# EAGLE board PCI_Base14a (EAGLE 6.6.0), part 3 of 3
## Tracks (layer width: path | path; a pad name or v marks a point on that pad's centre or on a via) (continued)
V33  (via drill 0.3) (continued)
  Top 0.152: C14.1 76.99,5.54 83.34,11.89 83.66,11.89 | R4.2 59.21,24.59 65.72,31.1 74.77,31.1 X5.5
  Top 0.254: v47.94,82.06 47.62,82.38 v47.62,88.25 47.62,90.48 47.15,90.95 47.15,92.06 46.67,92.54 46.67,94.29 46.59,94.36 | v45.08,82.06 45.08,79.05 X2.A53 | 46.59,94.36 45.08,95.87 45.08,96.67 X2.A39 | v46.67,103.49 v46.67,101.11 46.67,94.44 46.59,94.36 | v55.72,100.95 55.72,104.92 57.63,106.83 58.42,106.83 58.74,107.14 59.21,107.14 59.37,106.99 60.48,106.99 X1.B31 | v49.69,111.11 50.01,110.8 v50.01,100.95 | v50.96,118.73 50.96,111.43 v51.28,111.11 | v14.45,77.62 v14.45,91.59 v14.45,100.48 14.45,103.33 14.76,103.65 14.76,110 14.45,110.32 v14.45,114.45 | X3.B41 19.37,94.13 19.37,91.75 X3.B43 | X3.A53 24.45,79.05 24.45,80.79 26.03,82.38 v26.03,88.25 26.51,88.73 26.51,93.33 26.03,93.81 26.03,97.62 | 20.64,111.59 20.64,112.38 19.37,113.65 19.37,114.45 X3.B25 | 20.64,111.59 20.64,108.89 19.37,107.62 19.37,106.99 X3.B31 | 26.03,97.62 24.76,97.62 24.45,97.3 24.45,96.83 X3.A39 | 26.03,103.49 26.03,97.62 | v33.5,103.49 v33.5,100.48 | 26.03,103.49 26.19,103.65 26.19,110.95 v25.88,111.27 26.19,111.11 26.19,115.4 26.03,115.56 v26.03,118.73 | 26.03,103.49 v25.88,103.65 | X2.B25 40,114.45 40,113.65 38.73,112.38 38.73,108.89 40,107.62 40,106.99 X2.B31 40,106.83 40,106.03 38.73,104.76 38.73,102.54 37.46,101.27 37.46,100.64 X2.B36 37.46,100.48 37.46,99.68 38.73,98.41 38.73,96.19 40,94.92 40,94.29 X2.B41 40,94.13 40,91.75 X2.B43 40,91.59 40,91.27 41.75,91.27 42.07,91.59 43.02,91.59 43.34,91.27 43.5,91.27 45.08,89.68 45.08,89.21 X2.A45 | 20.64,111.59 21.11,111.59 21.43,111.91 22.38,111.91 22.7,112.22 24.45,112.22 24.45,112.07 X3.A27 | 83.66,9.83 X7.1 | 83.66,13.96 X7.2
  Top 0.254: v80.96,13.96 v80.96,31.26 80.96,52.38 v81.28,52.69 | v96.84,119.21 v96.84,116.19 96.52,115.88 v96.52,109.21 v96.52,108.26 96.52,101.43 v96.88,101.15 | v80.8,101.11 80.8,105.91 v81.12,106.23 | v85.09,119.21 85.09,118.57 84.93,118.42 84.93,114.61 v85.25,114.21 84.93,114.45 84.93,111.59 v85.25,111.27 | 67.87,103.73 67.63,103.97 v67.63,104.29 | 67.87,103.73 68.1,103.49 v68.1,96.67 68.42,96.67 68.42,89.36 v68.26,89.05 | v67.31,119.53 v67.31,111.91 67.31,109.84 67.94,109.21 67.94,103.81 67.87,103.73 | X1.B41 60.64,94.13 60.64,91.75 X1.B43 60.64,91.59 60.64,90.79 62.07,89.36 v62.07,89.21 | v74.77,89.05 74.77,84.28 JP1.1 | v73.34,84.13 v73.34,78.89 v73.34,75.08 v73.34,62.85 | v83.03,62.54 83.34,62.22 83.34,59.36 83.82,58.88 C10.+ 83.82,57.77 v83.82,52.69 | X1.B54 58.1,77.62 58.1,77.14 60.17,75.08 60.96,75.08 61.91,76.03 62.39,76.03 62.71,76.35 63.5,76.35 65.72,78.57 65.72,78.89 X1.A53
  Top 0.813: 83.66,13.96 83.66,11.89 83.66,9.83
  Bottom 0.152: X6.J3-D8 87.36,101.11 v80.8,101.11 | X6.J3-A17 arc90 X6.J3-A17 v96.84,119.21 | X6.J3-A12 arc90 X6.J3-A12 v96.52,109.21 | X6.J3-B11 91.99,108.02 arc-90 92.55,108.26 v96.52,108.26 | X6.J3-A8 arc90 93.46,101.11 v96.88,101.15 | X6.J3-C14 89.36,114.03 arc19 88.87,114.12 arc71 88.63,114.21 v85.25,114.21 | X6.J3-C10 89.36,105.94 arc19 89.35,106.02 arc71 89.11,106.19 81.28,106.23 | X6.J3-D17 arc-90 X6.J3-D17 v85.09,119.21 | X6.J3-B15 91.36,115.94 arc-90 91.61,116.19 v96.84,116.19
  Bottom 0.203: X6.J3-D13 85.25,111.21 80.01,111.21 80.01,111.27
  Bottom 0.254: X2.A53 45.08,78.89 46.04,78.89 47.78,77.14 56.67,77.14 57.15,77.62 57.94,77.62 X1.B54 | v47.62,88.25 47.31,88.57 46.51,88.57 46.04,89.05 45.08,89.05 X2.A45 | v45.08,82.06 v47.94,82.06 | v46.67,103.49 46.67,103.65 46.04,104.29 45.08,104.29 X2.A33 | 55.8,101.03 55.56,101.27 51.59,101.27 51.43,101.11 51.28,101.11 51.12,101.27 50.01,101.27 | 55.8,101.03 56.36,100.48 57.94,100.48 X1.B36 | 50.01,101.27 46.83,101.27 v46.67,101.11 | v55.72,100.95 55.8,101.03 | 50.01,101.27 v50.01,100.95 | X2.A27 45.08,111.91 46.04,111.91 46.51,111.43 49.37,111.43 v49.69,111.11 v51.28,111.11 | v50.96,118.73 50.64,119.05 46.51,119.05 46.04,119.53 45.08,119.53 X2.A21 | v14.45,77.62 16.67,77.62 X3.B54 | v14.45,91.59 19.21,91.59 X3.B43 | v14.45,100.48 16.67,100.48 X3.B36 | X3.A53 24.45,78.89 25.4,78.89 25.88,78.41 35.4,78.41 36.19,77.62 37.31,77.62 X2.B54 | v26.03,88.25 26.03,88.41 25.4,89.05 24.45,89.05 X3.A45 | 25.88,103.81 25.4,104.29 24.45,104.29 X3.A33 | v33.5,100.48 37.31,100.48 X2.B36 | v33.5,103.49 33.18,103.81 25.88,103.81 | 25.88,103.81 v25.88,103.65 | v25.88,111.27 25.88,111.43 25.4,111.91 24.45,111.91 X3.A27 | v26.03,118.73 26.03,118.89 25.4,119.53 24.45,119.53 X3.A21 | v14.45,114.45 19.21,114.45 X3.B25 | 74.93,31.26 X5.5 | 83.5,13.96 X7.2 | 89.06,9.83 X7.11 | 83.66,9.83 X7.1 | X6.J3-B15 91.28,115.08 90.96,114.76 90.49,114.76 89.85,114.13 89.38,114.13 88.87,114.12 | X6.J3-B11 91.28,107.14 90.8,107.14 89.69,106.03 89.38,106.03 89.35,106.02 | 81.28,106.23 v81.12,106.23 | v85.25,111.27 85.25,111.21 | v68.1,96.67 65.72,96.67 X1.A39 | v67.63,104.29 65.72,104.29 X1.A33 | v67.31,119.53 65.72,119.53 X1.A21
  Bottom 0.254: X1.B25 60.64,114.45 61.12,114.45 61.59,113.97 61.59,112.7 61.91,112.7 62.71,111.91 65.56,111.91 X1.A27 65.72,111.91 v67.31,111.91 67.79,111.43 73.5,111.43 73.82,111.75 79.53,111.75 80.01,111.27 | v74.77,89.05 v68.26,89.05 65.72,89.05 X1.A45 65.56,89.05 62.71,89.05 62.55,89.21 v62.07,89.21 | v73.34,75.08 74.93,75.08 JP3.1 | v73.34,84.13 74.77,84.13 JP1.1 | v83.03,62.54 73.66,62.54 v73.34,62.85 | v73.34,78.89 65.72,78.89 X1.A53 | v83.82,52.69 v81.28,52.69
  Bottom 0.813: v80.96,31.26 74.93,31.26 | 83.5,13.96 v80.96,13.96 | 83.66,9.83 89.06,9.83
V33IO  (via drill 0.3)
  Top 0.254: v73.02,113.97 73.02,115.56 C16.1 | v77.31,113.97 77.31,84.28 JP1.2
  Bottom 0.254: v77.31,113.97 v73.02,113.97
VIO  (via drill 0.3)
  Top 0.254: v83.03,124.25 v83.03,131.12 83.03,138.58 83.34,138.89 83.34,144.61 83.03,144.93 v83.03,147.47 | v95.57,136.2 v95.57,147.31 | v29.05,65.08 29.05,63.65 R6.2 | v49.37,65.08 49.37,63.65 R5.2 | JP3.2 77.63,74.92 77.63,72.54 JP3.4 77.63,72.38 v77.63,65.87 | v98.42,75.08 98.42,79.36 C17.1 98.42,79.52 v98.42,89.05 v98.42,98.25 | v97.63,136.2 97.31,135.88 97.31,129.69 97.63,129.37 97.63,127.78 96.04,126.19 96.04,111.43 95.73,111.11 95.73,106.19 96.04,105.87 96.04,98.57 v96.36,98.17
  Bottom 0.152: X6.J3-B6 92.51,98.21 v96.36,98.17 v98.42,98.25 | X6.J3-A2 X6.J3-A2 arc90 93.52,89.05 v98.42,89.05 | X6.J3-B25 91.36,136.2 v95.57,136.2 v97.63,136.2 | X6.J3-C19 89.36,123.88 arc90 88.43,124.21 v83.03,124.25 | X6.J3-D23 arc-90 87.27,131.12 v83.03,131.12
  Bottom 0.254: v83.03,147.47 83.18,147.31 v95.57,147.31 | v29.05,65.08 v49.37,65.08 50.16,65.87 v77.63,65.87 | v98.42,75.08 77.63,75.08 JP3.2

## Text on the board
tPlace: SLOT2 | SLOT1 | SLOT3 | V33IO | V33 | V5IO | V5P | V33 | VIO | V5P | V33 | V5P | +3,3V | V12P | +5V | V12M | ON | +12V | GND | OFF | -12V | GND | PS_ON# | PCI-SLOT-ERWEITERUNG 14b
